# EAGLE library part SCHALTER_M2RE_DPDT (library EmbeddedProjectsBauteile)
Schalter 2xUM
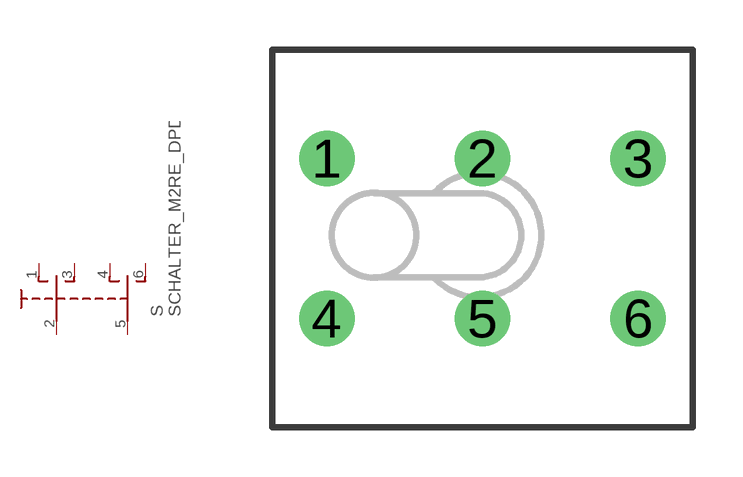
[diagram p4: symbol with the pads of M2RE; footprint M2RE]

Designator prefix S

## SCHALTER_M2RE_DPDT  [M2RE]
1  O  pas
2  P  pas
3  S  pas
4  O1  pas
5  P1  pas
6  S1  pas

## Footprint M2RE (pad centres in mm)
drill 1.1 pad 1.676: 1 -4.7,2.415; 2 0,2.415; 3 4.7,2.415; 4 -4.7,-2.415; 5 0,-2.415; 6 4.7,-2.415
